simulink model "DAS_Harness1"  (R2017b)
settings: Solver=FixedStepDiscrete  StartTime=0.0  StopTime=1  FixedStep=0.01  RelTol=1e-3  EnableMultiTasking=on
undefined symbols (not defined in the file): sigbuilder_block
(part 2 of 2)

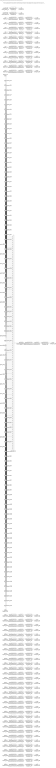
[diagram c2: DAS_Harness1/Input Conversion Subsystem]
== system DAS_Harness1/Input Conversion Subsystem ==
  note: This subsystem has been inserted by Simulink to adapt the output of the source blocks to the interface required by the harnessed component. Modifying the contents of this subsystem may result in compilation and simulation failure.
  Inport_1 : Inport
  Inport_2 : Inport  Port=2
  Inport_3 : Inport  Port=3
  Inport_4 : Inport  Port=4
  Inport_5 : Inport  Port=5
  Inport_6 : Inport  Port=6
  Inport_7 : Inport  Port=7
  Inport_8 : Inport  Port=8
  Inport_9 : Inport  Port=9
  Inport_10 : Inport  Port=10
  Inport_11 : Inport  Port=11
  Inport_12 : Inport  Port=12
  Inport_13 : Inport  Port=13
  Inport_14 : Inport  Port=14
  Inport_15 : Inport  Port=15
  Inport_16 : Inport  Port=16
  Inport_17 : Inport  Port=17
  Inport_18 : Inport  Port=18
  Inport_19 : Inport  Port=19
  Inport_20 : Inport  Port=20
  Inport_21 : Inport  Port=21
  Inport_22 : Inport  Port=22
  Inport_23 : Inport  Port=23
  Inport_24 : Inport  Port=24
  Inport_25 : Inport  Port=25
  Inport_26 : Inport  Port=26
  Inport_27 : Inport  Port=27
  Inport_28 : Inport  Port=28
  Inport_29 : Inport  Port=29
  Inport_30 : Inport  Port=30
  Inport_31 : Inport  Port=31
  Inport_32 : Inport  Port=32
  Inport_33 : Inport  Port=33
  Inport_34 : Inport  Port=34
  Inport_35 : Inport  Port=35
  Inport_36 : Inport  Port=36
  Inport_37 : Inport  Port=37
  Inport_38 : Inport  Port=38
  Inport_39 : Inport  Port=39
  Inport_40 : Inport  Port=40
  Inport_41 : Inport  Port=41
  Inport_42 : Inport  Port=42
  Inport_43 : Inport  Port=43
  Inport_44 : Inport  Port=44
  Inport_45 : Inport  Port=45
  Inport_46 : Inport  Port=46
  Inport_47 : Inport  Port=47
  Inport_48 : Inport  Port=48
  Inport_49 : Inport  Port=49
  Inport_50 : Inport  Port=50
  Inport_51 : Inport  Port=51
  Inport_52 : Inport  Port=52
  Inport_53 : Inport  Port=53
  Inport_54 : Inport  Port=54
  Inport_55 : Inport  Port=55
  Inport_56 : Inport  Port=56
  Inport_57 : Inport  Port=57
  Inport_58 : Inport  Port=58
  Inport_59 : Inport  Port=59
  Inport_60 : Inport  Port=60
  Inport_61 : Inport  Port=61
  Inport_62 : Inport  Port=62
  Inport_63 : Inport  Port=63
  Inport_64 : Inport  Port=64
  Inport_65 : Inport  Port=65
  Inport_66 : Inport  Port=66
  Inport_67 : Inport  Port=67
  Inport_68 : Inport  Port=68
  Inport_69 : Inport  Port=69
  Inport_70 : Inport  Port=70
  Inport_71 : Inport  Port=71
  Inport_72 : Inport  Port=72
  Inport_73 : Inport  Port=73
  Inport_74 : Inport  Port=74
  Inport_75 : Inport  Port=75
  Inport_76 : Inport  Port=76
  Inport_77 : Inport  Port=77
  Inport_78 : Inport  Port=78
  Inport_79 : Inport  Port=79
  Inport_80 : Inport  Port=80
  Inport_81 : Inport  Port=81
  Inport_82 : Inport  Port=82
  Inport_83 : Inport  Port=83
  Inport_84 : Inport  Port=84
  Inport_85 : Inport  Port=85
  Inport_86 : Inport  Port=86
  Inport_87 : Inport  Port=87
  Inport_88 : Inport  Port=88
  Inport_89 : Inport  Port=89
  Inport_90 : Inport  Port=90
  Inport_91 : Inport  Port=91
  Inport_92 : Inport  Port=92
  Inport_93 : Inport  Port=93
  Inport_94 : Inport  Port=94
  Inport_95 : Inport  Port=95
  Inport_96 : Inport  Port=96
  Inport_97 : Inport  Port=97
  Inport_98 : Inport  Port=98
  Inport_99 : Inport  Port=99
  Inport_100 : Inport  Port=100
  Inport_101 : Inport  Port=101
  Inport_102 : Inport  Port=102
  Inport_103 : Inport  Port=103
  Inport_104 : Inport  Port=104
  Inport_105 : Inport  Port=105
  Inport_106 : Inport  Port=106
  Inport_107 : Inport  Port=107
  Inport_108 : Inport  Port=108
  Inport_109 : Inport  Port=109
  Inport_110 : Inport  Port=110
  Inport_111 : Inport  Port=111
  Inport_112 : Inport  Port=112
  Inport_113 : Inport  Port=113
  Inport_114 : Inport  Port=114
  Inport_115 : Inport  Port=115
  Inport_116 : Inport  Port=116
  Inport_117 : Inport  Port=117
  Inport_118 : Inport  Port=118
  Inport_119 : Inport  Port=119
  Inport_120 : Inport  Port=120
  Inport_121 : Inport  Port=121
  Inport_122 : Inport  Port=122
  Inport_123 : Inport  Port=123
  Inport_124 : Inport  Port=124
  Inport_125 : Inport  Port=125
  Inport_126 : Inport  Port=126
  Inport_127 : Inport  Port=127
  Inport_128 : Inport  Port=128
  Inport_129 : Inport  Port=129
  Inport_130 : Inport  Port=130
  Inport_131 : Inport  Port=131
  Inport_132 : Inport  Port=132
  Inport_133 : Inport  Port=133
  Inport_134 : Inport  Port=134
  Inport_135 : Inport  Port=135
  Inport_136 : Inport  Port=136
  Inport_137 : Inport  Port=137
  Inport_138 : Inport  Port=138
  Inport_139 : Inport  Port=139
  Inport_140 : Inport  Port=140
  Inport_141 : Inport  Port=141
  Inport_142 : Inport  Port=142
  Inport_143 : Inport  Port=143
  Inport_144 : Inport  Port=144
  Inport_145 : Inport  Port=145
  Inport_146 : Inport  Port=146
  Inport_147 : Inport  Port=147
  Inport_148 : Inport  Port=148
  Inport_149 : Inport  Port=149
  Inport_150 : Inport  Port=150
  Inport_151 : Inport  Port=151
  Inport_152 : Inport  Port=152
  Inport_153 : Inport  Port=153
  Inport_154 : Inport  Port=154
  Inport_155 : Inport  Port=155
  Inport_156 : Inport  Port=156
  Concat_1 : Concatenate  NumInputs=112
  Data_Conversion_{1..2,12,15..18} (7 alike) : DataTypeConversion  OutDataTypeStr=single
  Data_Conversion_{3..11,13,19..28,30..46} (37 alike) : DataTypeConversion  OutDataTypeStr=boolean
  Data_Conversion_14 : Reshape  OutputDimensionality=Customize  OutputDimensions=[112]
  Data_Conversion_29 : DataTypeConversion  OutDataTypeStr=uint8
  RateTs_{1..45} (45 alike) : RateTransition
  SigSpec_1 : SignalSpecification
  SigSpec_{6..13,36} (9 alike) : SignalSpecification  OutDataTypeStr=boolean  Unit=flg  Dimensions=[1]
  SigSpec_14 : SignalSpecification  OutDataTypeStr=single  Unit=A  Dimensions=[1]
  SigSpec_15 : SignalSpecification  OutDataTypeStr=boolean  Unit=flag  Dimensions=[112]
  SigSpec_{16..19} (4 alike) : SignalSpecification  OutDataTypeStr=single  Unit=pct  Dimensions=[1]
  SigSpec_2 : SignalSpecification
  SigSpec_{5,20..29,31..35,37..47} (27 alike) : SignalSpecification  OutDataTypeStr=boolean  Unit=flag  Dimensions=[1]
  SigSpec_3 : SignalSpecification  OutDataTypeStr=single  Unit=C  Dimensions=[1]
  SigSpec_30 : SignalSpecification  OutDataTypeStr=uint8  Unit=enum  Dimensions=[1]
  SigSpec_4 : SignalSpecification  OutDataTypeStr=single  Unit=C  Dimensions=[1]
  Outport_1 : Outport
  Outport_2 : Outport  Port=2
  Outport_3 : Outport  Port=3
  Outport_4 : Outport  Port=4
  Outport_5 : Outport  Port=5
  Outport_6 : Outport  Port=6
  Outport_7 : Outport  Port=7
  Outport_8 : Outport  Port=8
  Outport_9 : Outport  Port=9
  Outport_10 : Outport  Port=10
  Outport_11 : Outport  Port=11
  Outport_12 : Outport  Port=12
  Outport_13 : Outport  Port=13
  Outport_14 : Outport  Port=14
  Outport_15 : Outport  Port=15
  Outport_16 : Outport  Port=16
  Outport_17 : Outport  Port=17
  Outport_18 : Outport  Port=18
  Outport_19 : Outport  Port=19
  Outport_20 : Outport  Port=20
  Outport_21 : Outport  Port=21
  Outport_22 : Outport  Port=22
  Outport_23 : Outport  Port=23
  Outport_24 : Outport  Port=24
  Outport_25 : Outport  Port=25
  Outport_26 : Outport  Port=26
  Outport_27 : Outport  Port=27
  Outport_28 : Outport  Port=28
  Outport_29 : Outport  Port=29
  Outport_30 : Outport  Port=30
  Outport_31 : Outport  Port=31
  Outport_32 : Outport  Port=32
  Outport_33 : Outport  Port=33
  Outport_34 : Outport  Port=34
  Outport_35 : Outport  Port=35
  Outport_36 : Outport  Port=36
  Outport_37 : Outport  Port=37
  Outport_38 : Outport  Port=38
  Outport_39 : Outport  Port=39
  Outport_40 : Outport  Port=40
  Outport_41 : Outport  Port=41
  Outport_42 : Outport  Port=42
  Outport_43 : Outport  Port=43
  Outport_44 : Outport  Port=44
  Outport_45 : Outport  Port=45
  Outport_46 : Outport  Port=46
  Outport_47 : Outport  Port=47
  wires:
  SigSpec_1/1 -> Outport_1/1
  [send_fcn1] -> SigSpec_1/1
  SigSpec_2/1 -> Outport_2/1
  [send_fcn2] -> SigSpec_2/1
  SigSpec_3/1 -> Outport_3/1
  RateTs_1/1 -> SigSpec_3/1
  Data_Conversion_1/1 -> RateTs_1/1
  Inport_1/1 -> Data_Conversion_1/1
  SigSpec_4/1 -> Outport_4/1
  RateTs_2/1 -> SigSpec_4/1
  Data_Conversion_2/1 -> RateTs_2/1
  Inport_2/1 -> Data_Conversion_2/1
  SigSpec_5/1 -> Outport_5/1
  RateTs_3/1 -> SigSpec_5/1
  Data_Conversion_3/1 -> RateTs_3/1
  Inport_3/1 -> Data_Conversion_3/1
  SigSpec_6/1 -> Outport_6/1
  RateTs_4/1 -> SigSpec_6/1
  Data_Conversion_4/1 -> RateTs_4/1
  Inport_4/1 -> Data_Conversion_4/1
  SigSpec_7/1 -> Outport_7/1
  RateTs_5/1 -> SigSpec_7/1
  Data_Conversion_5/1 -> RateTs_5/1
  Inport_5/1 -> Data_Conversion_5/1
  SigSpec_8/1 -> Outport_8/1
  RateTs_6/1 -> SigSpec_8/1
  Data_Conversion_6/1 -> RateTs_6/1
  Inport_6/1 -> Data_Conversion_6/1
  SigSpec_9/1 -> Outport_9/1
  RateTs_7/1 -> SigSpec_9/1
  Data_Conversion_7/1 -> RateTs_7/1
  Inport_7/1 -> Data_Conversion_7/1
  SigSpec_10/1 -> Outport_10/1
  RateTs_8/1 -> SigSpec_10/1
  Data_Conversion_8/1 -> RateTs_8/1
  Inport_8/1 -> Data_Conversion_8/1
  SigSpec_11/1 -> Outport_11/1
  RateTs_9/1 -> SigSpec_11/1
  Data_Conversion_9/1 -> RateTs_9/1
  Inport_9/1 -> Data_Conversion_9/1
  SigSpec_12/1 -> Outport_12/1
  RateTs_10/1 -> SigSpec_12/1
  Data_Conversion_10/1 -> RateTs_10/1
  Inport_10/1 -> Data_Conversion_10/1
  SigSpec_13/1 -> Outport_13/1
  RateTs_11/1 -> SigSpec_13/1
  Data_Conversion_11/1 -> RateTs_11/1
  Inport_11/1 -> Data_Conversion_11/1
  SigSpec_14/1 -> Outport_14/1
  RateTs_12/1 -> SigSpec_14/1
  Data_Conversion_12/1 -> RateTs_12/1
  Inport_12/1 -> Data_Conversion_12/1
  SigSpec_15/1 -> Outport_15/1
  RateTs_13/1 -> SigSpec_15/1
  Data_Conversion_13/1 -> RateTs_13/1
  Data_Conversion_14/1 -> Data_Conversion_13/1
  Concat_1/1 -> Data_Conversion_14/1
  Inport_13/1 -> Concat_1/1
  Inport_14/1 -> Concat_1/2
  Inport_15/1 -> Concat_1/3
  Inport_16/1 -> Concat_1/4
  Inport_17/1 -> Concat_1/5
  Inport_18/1 -> Concat_1/6
  Inport_19/1 -> Concat_1/7
  Inport_20/1 -> Concat_1/8
  Inport_21/1 -> Concat_1/9
  Inport_22/1 -> Concat_1/10
  Inport_23/1 -> Concat_1/11
  Inport_24/1 -> Concat_1/12
  Inport_25/1 -> Concat_1/13
  Inport_26/1 -> Concat_1/14
  Inport_27/1 -> Concat_1/15
  Inport_28/1 -> Concat_1/16
  Inport_29/1 -> Concat_1/17
  Inport_30/1 -> Concat_1/18
  Inport_31/1 -> Concat_1/19
  Inport_32/1 -> Concat_1/20
  Inport_33/1 -> Concat_1/21
  Inport_34/1 -> Concat_1/22
  Inport_35/1 -> Concat_1/23
  Inport_36/1 -> Concat_1/24
  Inport_37/1 -> Concat_1/25
  Inport_38/1 -> Concat_1/26
  Inport_39/1 -> Concat_1/27
  Inport_40/1 -> Concat_1/28
  Inport_41/1 -> Concat_1/29
  Inport_42/1 -> Concat_1/30
  Inport_43/1 -> Concat_1/31
  Inport_44/1 -> Concat_1/32
  Inport_45/1 -> Concat_1/33
  Inport_46/1 -> Concat_1/34
  Inport_47/1 -> Concat_1/35
  Inport_48/1 -> Concat_1/36
  Inport_49/1 -> Concat_1/37
  Inport_50/1 -> Concat_1/38
  Inport_51/1 -> Concat_1/39
  Inport_52/1 -> Concat_1/40
  Inport_53/1 -> Concat_1/41
  Inport_54/1 -> Concat_1/42
  Inport_55/1 -> Concat_1/43
  Inport_56/1 -> Concat_1/44
  Inport_57/1 -> Concat_1/45
  Inport_58/1 -> Concat_1/46
  Inport_59/1 -> Concat_1/47
  Inport_60/1 -> Concat_1/48
  Inport_61/1 -> Concat_1/49
  Inport_62/1 -> Concat_1/50
  Inport_63/1 -> Concat_1/51
  Inport_64/1 -> Concat_1/52
  Inport_65/1 -> Concat_1/53
  Inport_66/1 -> Concat_1/54
  Inport_67/1 -> Concat_1/55
  Inport_68/1 -> Concat_1/56
  Inport_69/1 -> Concat_1/57
  Inport_70/1 -> Concat_1/58
  Inport_71/1 -> Concat_1/59
  Inport_72/1 -> Concat_1/60
  Inport_73/1 -> Concat_1/61
  Inport_74/1 -> Concat_1/62
  Inport_75/1 -> Concat_1/63
  Inport_76/1 -> Concat_1/64
  Inport_77/1 -> Concat_1/65
  Inport_78/1 -> Concat_1/66
  Inport_79/1 -> Concat_1/67
  Inport_80/1 -> Concat_1/68
  Inport_81/1 -> Concat_1/69
  Inport_82/1 -> Concat_1/70
  Inport_83/1 -> Concat_1/71
  Inport_84/1 -> Concat_1/72
  Inport_85/1 -> Concat_1/73
  Inport_86/1 -> Concat_1/74
  Inport_87/1 -> Concat_1/75
  Inport_88/1 -> Concat_1/76
  Inport_89/1 -> Concat_1/77
  Inport_90/1 -> Concat_1/78
  Inport_91/1 -> Concat_1/79
  Inport_92/1 -> Concat_1/80
  Inport_93/1 -> Concat_1/81
  Inport_94/1 -> Concat_1/82
  Inport_95/1 -> Concat_1/83
  Inport_96/1 -> Concat_1/84
  Inport_97/1 -> Concat_1/85
  Inport_98/1 -> Concat_1/86
  Inport_99/1 -> Concat_1/87
  Inport_100/1 -> Concat_1/88
  Inport_101/1 -> Concat_1/89
  Inport_102/1 -> Concat_1/90
  Inport_103/1 -> Concat_1/91
  Inport_104/1 -> Concat_1/92
  Inport_105/1 -> Concat_1/93
  Inport_106/1 -> Concat_1/94
  Inport_107/1 -> Concat_1/95
  Inport_108/1 -> Concat_1/96
  Inport_109/1 -> Concat_1/97
  Inport_110/1 -> Concat_1/98
  Inport_111/1 -> Concat_1/99
  Inport_112/1 -> Concat_1/100
  Inport_113/1 -> Concat_1/101
  Inport_114/1 -> Concat_1/102
  Inport_115/1 -> Concat_1/103
  Inport_116/1 -> Concat_1/104
  Inport_117/1 -> Concat_1/105
  Inport_118/1 -> Concat_1/106
  Inport_119/1 -> Concat_1/107
  Inport_120/1 -> Concat_1/108
  Inport_121/1 -> Concat_1/109
  Inport_122/1 -> Concat_1/110
  Inport_123/1 -> Concat_1/111
  Inport_124/1 -> Concat_1/112
  SigSpec_16/1 -> Outport_16/1
  RateTs_14/1 -> SigSpec_16/1
  Data_Conversion_15/1 -> RateTs_14/1
  Inport_125/1 -> Data_Conversion_15/1
  SigSpec_17/1 -> Outport_17/1
  RateTs_15/1 -> SigSpec_17/1
  Data_Conversion_16/1 -> RateTs_15/1
  Inport_126/1 -> Data_Conversion_16/1
  SigSpec_18/1 -> Outport_18/1
  RateTs_16/1 -> SigSpec_18/1
  Data_Conversion_17/1 -> RateTs_16/1
  Inport_127/1 -> Data_Conversion_17/1
  SigSpec_19/1 -> Outport_19/1
  RateTs_17/1 -> SigSpec_19/1
  Data_Conversion_18/1 -> RateTs_17/1
  Inport_128/1 -> Data_Conversion_18/1
  SigSpec_20/1 -> Outport_20/1
  RateTs_18/1 -> SigSpec_20/1
  Data_Conversion_19/1 -> RateTs_18/1
  Inport_129/1 -> Data_Conversion_19/1
  SigSpec_21/1 -> Outport_21/1
  RateTs_19/1 -> SigSpec_21/1
  Data_Conversion_20/1 -> RateTs_19/1
  Inport_130/1 -> Data_Conversion_20/1
  SigSpec_22/1 -> Outport_22/1
  RateTs_20/1 -> SigSpec_22/1
  Data_Conversion_21/1 -> RateTs_20/1
  Inport_131/1 -> Data_Conversion_21/1
  SigSpec_23/1 -> Outport_23/1
  RateTs_21/1 -> SigSpec_23/1
  Data_Conversion_22/1 -> RateTs_21/1
  Inport_132/1 -> Data_Conversion_22/1
  SigSpec_24/1 -> Outport_24/1
  RateTs_22/1 -> SigSpec_24/1
  Data_Conversion_23/1 -> RateTs_22/1
  Inport_133/1 -> Data_Conversion_23/1
  SigSpec_25/1 -> Outport_25/1
  RateTs_23/1 -> SigSpec_25/1
  Data_Conversion_24/1 -> RateTs_23/1
  Inport_134/1 -> Data_Conversion_24/1
  SigSpec_26/1 -> Outport_26/1
  RateTs_24/1 -> SigSpec_26/1
  Data_Conversion_25/1 -> RateTs_24/1
  Inport_135/1 -> Data_Conversion_25/1
  SigSpec_27/1 -> Outport_27/1
  RateTs_25/1 -> SigSpec_27/1
  Data_Conversion_26/1 -> RateTs_25/1
  Inport_136/1 -> Data_Conversion_26/1
  SigSpec_28/1 -> Outport_28/1
  RateTs_26/1 -> SigSpec_28/1
  Data_Conversion_27/1 -> RateTs_26/1
  Inport_137/1 -> Data_Conversion_27/1
  SigSpec_29/1 -> Outport_29/1
  RateTs_27/1 -> SigSpec_29/1
  Data_Conversion_28/1 -> RateTs_27/1
  Inport_138/1 -> Data_Conversion_28/1
  SigSpec_30/1 -> Outport_30/1
  RateTs_28/1 -> SigSpec_30/1
  Data_Conversion_29/1 -> RateTs_28/1
  Inport_139/1 -> Data_Conversion_29/1
  SigSpec_31/1 -> Outport_31/1
  RateTs_29/1 -> SigSpec_31/1
  Data_Conversion_30/1 -> RateTs_29/1
  Inport_140/1 -> Data_Conversion_30/1
  SigSpec_32/1 -> Outport_32/1
  RateTs_30/1 -> SigSpec_32/1
  Data_Conversion_31/1 -> RateTs_30/1
  Inport_141/1 -> Data_Conversion_31/1
  SigSpec_33/1 -> Outport_33/1
  RateTs_31/1 -> SigSpec_33/1
  Data_Conversion_32/1 -> RateTs_31/1
  Inport_142/1 -> Data_Conversion_32/1
  SigSpec_34/1 -> Outport_34/1
  RateTs_32/1 -> SigSpec_34/1
  Data_Conversion_33/1 -> RateTs_32/1
  Inport_143/1 -> Data_Conversion_33/1
  SigSpec_35/1 -> Outport_35/1
  RateTs_33/1 -> SigSpec_35/1
  Data_Conversion_34/1 -> RateTs_33/1
  Inport_144/1 -> Data_Conversion_34/1
  SigSpec_36/1 -> Outport_36/1
  RateTs_34/1 -> SigSpec_36/1
  Data_Conversion_35/1 -> RateTs_34/1
  Inport_145/1 -> Data_Conversion_35/1
  SigSpec_37/1 -> Outport_37/1
  RateTs_35/1 -> SigSpec_37/1
  Data_Conversion_36/1 -> RateTs_35/1
  Inport_146/1 -> Data_Conversion_36/1
  SigSpec_38/1 -> Outport_38/1
  RateTs_36/1 -> SigSpec_38/1
  Data_Conversion_37/1 -> RateTs_36/1
  Inport_147/1 -> Data_Conversion_37/1
  SigSpec_39/1 -> Outport_39/1
  RateTs_37/1 -> SigSpec_39/1
  Data_Conversion_38/1 -> RateTs_37/1
  Inport_148/1 -> Data_Conversion_38/1
  SigSpec_40/1 -> Outport_40/1
  RateTs_38/1 -> SigSpec_40/1
  Data_Conversion_39/1 -> RateTs_38/1
  Inport_149/1 -> Data_Conversion_39/1
  SigSpec_41/1 -> Outport_41/1
  RateTs_39/1 -> SigSpec_41/1
  Data_Conversion_40/1 -> RateTs_39/1
  Inport_150/1 -> Data_Conversion_40/1
  SigSpec_42/1 -> Outport_42/1
  RateTs_40/1 -> SigSpec_42/1
  Data_Conversion_41/1 -> RateTs_40/1
  Inport_151/1 -> Data_Conversion_41/1
  SigSpec_43/1 -> Outport_43/1
  RateTs_41/1 -> SigSpec_43/1
  Data_Conversion_42/1 -> RateTs_41/1
  Inport_152/1 -> Data_Conversion_42/1
  SigSpec_44/1 -> Outport_44/1
  RateTs_42/1 -> SigSpec_44/1
  Data_Conversion_43/1 -> RateTs_42/1
  Inport_153/1 -> Data_Conversion_43/1
  SigSpec_45/1 -> Outport_45/1
  RateTs_43/1 -> SigSpec_45/1
  Data_Conversion_44/1 -> RateTs_43/1
  Inport_154/1 -> Data_Conversion_44/1
  SigSpec_46/1 -> Outport_46/1
  RateTs_44/1 -> SigSpec_46/1
  Data_Conversion_45/1 -> RateTs_44/1
  Inport_155/1 -> Data_Conversion_45/1
  SigSpec_47/1 -> Outport_47/1
  RateTs_45/1 -> SigSpec_47/1
  Data_Conversion_46/1 -> RateTs_45/1
  Inport_156/1 -> Data_Conversion_46/1

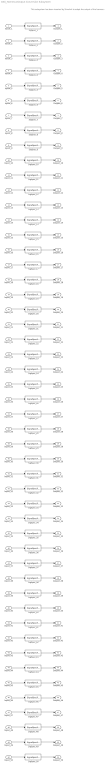
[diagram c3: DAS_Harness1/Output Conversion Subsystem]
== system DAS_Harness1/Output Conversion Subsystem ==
  note: This subsystem has been inserted by Simulink to adapt the output of the harnessed component to the interface required by the sink blocks. Modifying the contents of this subsystem may result in compilation and simulation failure.
  Inport_1 : Inport
  Inport_2 : Inport  Port=2
  Inport_3 : Inport  Port=3
  Inport_4 : Inport  Port=4
  Inport_5 : Inport  Port=5
  Inport_6 : Inport  Port=6
  Inport_7 : Inport  Port=7
  Inport_8 : Inport  Port=8
  Inport_9 : Inport  Port=9
  Inport_10 : Inport  Port=10
  Inport_11 : Inport  Port=11
  Inport_12 : Inport  Port=12
  Inport_13 : Inport  Port=13
  Inport_14 : Inport  Port=14
  Inport_15 : Inport  Port=15
  Inport_16 : Inport  Port=16
  Inport_17 : Inport  Port=17
  Inport_18 : Inport  Port=18
  Inport_19 : Inport  Port=19
  Inport_20 : Inport  Port=20
  Inport_21 : Inport  Port=21
  Inport_22 : Inport  Port=22
  Inport_23 : Inport  Port=23
  Inport_24 : Inport  Port=24
  Inport_25 : Inport  Port=25
  Inport_26 : Inport  Port=26
  Inport_27 : Inport  Port=27
  Inport_28 : Inport  Port=28
  Inport_29 : Inport  Port=29
  Inport_30 : Inport  Port=30
  Inport_31 : Inport  Port=31
  Inport_32 : Inport  Port=32
  Inport_33 : Inport  Port=33
  Inport_34 : Inport  Port=34
  Inport_35 : Inport  Port=35
  Inport_36 : Inport  Port=36
  Inport_37 : Inport  Port=37
  Inport_38 : Inport  Port=38
  Inport_39 : Inport  Port=39
  Inport_40 : Inport  Port=40
  Inport_41 : Inport  Port=41
  Inport_42 : Inport  Port=42
  Inport_43 : Inport  Port=43
  Inport_44 : Inport  Port=44
  Inport_45 : Inport  Port=45
  Inport_46 : Inport  Port=46
  Inport_47 : Inport  Port=47
  Inport_48 : Inport  Port=48
  Inport_49 : Inport  Port=49
  Inport_50 : Inport  Port=50
  SigSpec_{1..6,8,17..29,34..35,40..48} (31 alike) : SignalSpecification  OutDataTypeStr=uint16  Unit=numb  Dimensions=[1]
  SigSpec_{9..16,30..33,36..39} (16 alike) : SignalSpecification  OutDataTypeStr=single  Unit=min  Dimensions=[1]
  SigSpec_49 : SignalSpecification  OutDataTypeStr=boolean  Unit=numb  Dimensions=[1]
  SigSpec_50 : SignalSpecification  OutDataTypeStr=boolean  Unit=numb  Dimensions=[1]
  SigSpec_7 : SignalSpecification  OutDataTypeStr=uint32  Unit=numb  Dimensions=[1]
  Outport_1 : Outport
  Outport_2 : Outport  Port=2
  Outport_3 : Outport  Port=3
  Outport_4 : Outport  Port=4
  Outport_5 : Outport  Port=5
  Outport_6 : Outport  Port=6
  Outport_7 : Outport  Port=7
  Outport_8 : Outport  Port=8
  Outport_9 : Outport  Port=9
  Outport_10 : Outport  Port=10
  Outport_11 : Outport  Port=11
  Outport_12 : Outport  Port=12
  Outport_13 : Outport  Port=13
  Outport_14 : Outport  Port=14
  Outport_15 : Outport  Port=15
  Outport_16 : Outport  Port=16
  Outport_17 : Outport  Port=17
  Outport_18 : Outport  Port=18
  Outport_19 : Outport  Port=19
  Outport_20 : Outport  Port=20
  Outport_21 : Outport  Port=21
  Outport_22 : Outport  Port=22
  Outport_23 : Outport  Port=23
  Outport_24 : Outport  Port=24
  Outport_25 : Outport  Port=25
  Outport_26 : Outport  Port=26
  Outport_27 : Outport  Port=27
  Outport_28 : Outport  Port=28
  Outport_29 : Outport  Port=29
  Outport_30 : Outport  Port=30
  Outport_31 : Outport  Port=31
  Outport_32 : Outport  Port=32
  Outport_33 : Outport  Port=33
  Outport_34 : Outport  Port=34
  Outport_35 : Outport  Port=35
  Outport_36 : Outport  Port=36
  Outport_37 : Outport  Port=37
  Outport_38 : Outport  Port=38
  Outport_39 : Outport  Port=39
  Outport_40 : Outport  Port=40
  Outport_41 : Outport  Port=41
  Outport_42 : Outport  Port=42
  Outport_43 : Outport  Port=43
  Outport_44 : Outport  Port=44
  Outport_45 : Outport  Port=45
  Outport_46 : Outport  Port=46
  Outport_47 : Outport  Port=47
  Outport_48 : Outport  Port=48
  Outport_49 : Outport  Port=49
  Outport_50 : Outport  Port=50
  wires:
  Inport_1/1 -> SigSpec_1/1
  SigSpec_1/1 -> Outport_1/1
  Inport_2/1 -> SigSpec_2/1
  SigSpec_2/1 -> Outport_2/1
  Inport_3/1 -> SigSpec_3/1
  SigSpec_3/1 -> Outport_3/1
  Inport_4/1 -> SigSpec_4/1
  SigSpec_4/1 -> Outport_4/1
  Inport_5/1 -> SigSpec_5/1
  SigSpec_5/1 -> Outport_5/1
  Inport_6/1 -> SigSpec_6/1
  SigSpec_6/1 -> Outport_6/1
  Inport_7/1 -> SigSpec_7/1
  SigSpec_7/1 -> Outport_7/1
  Inport_8/1 -> SigSpec_8/1
  SigSpec_8/1 -> Outport_8/1
  Inport_9/1 -> SigSpec_9/1
  SigSpec_9/1 -> Outport_9/1
  Inport_10/1 -> SigSpec_10/1
  SigSpec_10/1 -> Outport_10/1
  Inport_11/1 -> SigSpec_11/1
  SigSpec_11/1 -> Outport_11/1
  Inport_12/1 -> SigSpec_12/1
  SigSpec_12/1 -> Outport_12/1
  Inport_13/1 -> SigSpec_13/1
  SigSpec_13/1 -> Outport_13/1
  Inport_14/1 -> SigSpec_14/1
  SigSpec_14/1 -> Outport_14/1
  Inport_15/1 -> SigSpec_15/1
  SigSpec_15/1 -> Outport_15/1
  Inport_16/1 -> SigSpec_16/1
  SigSpec_16/1 -> Outport_16/1
  Inport_17/1 -> SigSpec_17/1
  SigSpec_17/1 -> Outport_17/1
  Inport_18/1 -> SigSpec_18/1
  SigSpec_18/1 -> Outport_18/1
  Inport_19/1 -> SigSpec_19/1
  SigSpec_19/1 -> Outport_19/1
  Inport_20/1 -> SigSpec_20/1
  SigSpec_20/1 -> Outport_20/1
  Inport_21/1 -> SigSpec_21/1
  SigSpec_21/1 -> Outport_21/1
  Inport_22/1 -> SigSpec_22/1
  SigSpec_22/1 -> Outport_22/1
  Inport_23/1 -> SigSpec_23/1
  SigSpec_23/1 -> Outport_23/1
  Inport_24/1 -> SigSpec_24/1
  SigSpec_24/1 -> Outport_24/1
  Inport_25/1 -> SigSpec_25/1
  SigSpec_25/1 -> Outport_25/1
  Inport_26/1 -> SigSpec_26/1
  SigSpec_26/1 -> Outport_26/1
  Inport_27/1 -> SigSpec_27/1
  SigSpec_27/1 -> Outport_27/1
  Inport_28/1 -> SigSpec_28/1
  SigSpec_28/1 -> Outport_28/1
  Inport_29/1 -> SigSpec_29/1
  SigSpec_29/1 -> Outport_29/1
  Inport_30/1 -> SigSpec_30/1
  SigSpec_30/1 -> Outport_30/1
  Inport_31/1 -> SigSpec_31/1
  SigSpec_31/1 -> Outport_31/1
  Inport_32/1 -> SigSpec_32/1
  SigSpec_32/1 -> Outport_32/1
  Inport_33/1 -> SigSpec_33/1
  SigSpec_33/1 -> Outport_33/1
  Inport_34/1 -> SigSpec_34/1
  SigSpec_34/1 -> Outport_34/1
  Inport_35/1 -> SigSpec_35/1
  SigSpec_35/1 -> Outport_35/1
  Inport_36/1 -> SigSpec_36/1
  SigSpec_36/1 -> Outport_36/1
  Inport_37/1 -> SigSpec_37/1
  SigSpec_37/1 -> Outport_37/1
  Inport_38/1 -> SigSpec_38/1
  SigSpec_38/1 -> Outport_38/1
  Inport_39/1 -> SigSpec_39/1
  SigSpec_39/1 -> Outport_39/1
  Inport_40/1 -> SigSpec_40/1
  SigSpec_40/1 -> Outport_40/1
  Inport_41/1 -> SigSpec_41/1
  SigSpec_41/1 -> Outport_41/1
  Inport_42/1 -> SigSpec_42/1
  SigSpec_42/1 -> Outport_42/1
  Inport_43/1 -> SigSpec_43/1
  SigSpec_43/1 -> Outport_43/1
  Inport_44/1 -> SigSpec_44/1
  SigSpec_44/1 -> Outport_44/1
  Inport_45/1 -> SigSpec_45/1
  SigSpec_45/1 -> Outport_45/1
  Inport_46/1 -> SigSpec_46/1
  SigSpec_46/1 -> Outport_46/1
  Inport_47/1 -> SigSpec_47/1
  SigSpec_47/1 -> Outport_47/1
  Inport_48/1 -> SigSpec_48/1
  SigSpec_48/1 -> Outport_48/1
  Inport_49/1 -> SigSpec_49/1
  SigSpec_49/1 -> Outport_49/1
  Inport_50/1 -> SigSpec_50/1
  SigSpec_50/1 -> Outport_50/1

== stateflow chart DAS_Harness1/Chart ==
  state Run
    en:
    Run10ms;
    Run100ms;
    Run -> (junction 1) : {Run10ms}
    (junction 1) -> (junction 3)
    (junction 3) -> (junction 5) : [i>8]
    (junction 3) -> (junction 9) : {i = i + 1}
    (junction 5) -> (junction 11) : {Run100ms}
    (junction 11) -> (junction 9) : {i=0}
    (junction 9) -> (junction 14)
  (default) -> Run
  data: i local =0
  events: output FUNCTION_CALL_EVENT; output FUNCTION_CALL_EVENT

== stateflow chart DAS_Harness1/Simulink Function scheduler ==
  state Run
  state AsyncFunctionCalls
    % Call Asynchronous FunctionCall Subsystems.
    %
    %% Schedule function-call outputs.
    %% Modify this code to change function-call order.
    send(DAS_DataFastAbsStr_10ms)
    send(DAS_DataSlowAbsStr_100ms)
  (default) -> Run
  events: output FUNCTION_CALL_EVENT; output FUNCTION_CALL_EVENT
